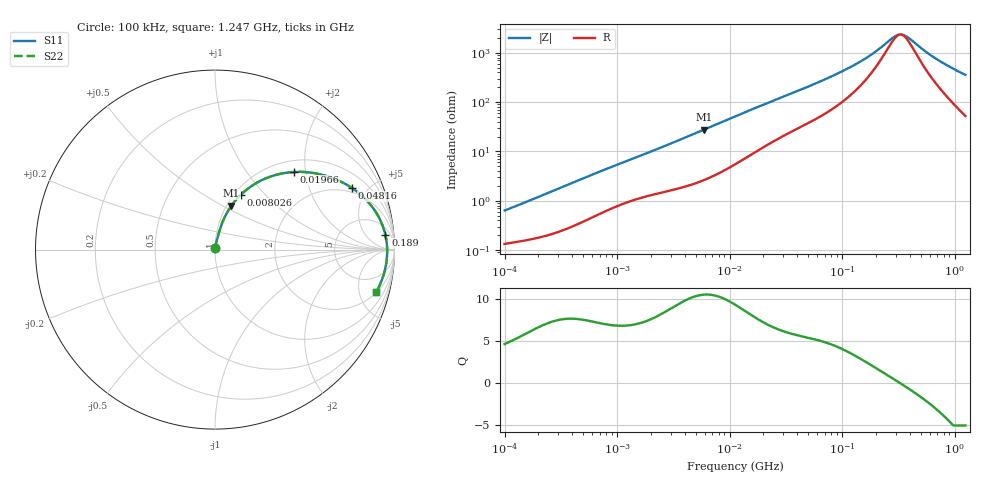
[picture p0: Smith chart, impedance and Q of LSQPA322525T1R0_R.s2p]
! LSQPA322525T1R0_R  S-PARAMETER MODEL  ( General Type )
! Model Generated by TAIYO YUDEN Corporation (http://www.ty-top.com)
! Version 2.0
! TAIYO YUDEN Control No. 100810NF25SB-FKC
! Copyright(c) 2007 TAIYO YUDEN CO.,LTD. All Rights Reserved.
! Product Description (link to TY-COMPAS)
! https://ds.yuden.co.jp/TYCOMPAS/or/detail?pn=LSQPA322525T1R0MR&u=M
! Products Name : Inductors
! Characteristics :
!  Inductance : 1.0 uH , SRF(min) : 250 MHz , DC Resistance(max) : 0.0715 Ohm
!  Rated Current : Saturation :2000 mA , Temp Rise : 1440 mA (40 degC)
!  Case Size : 3.2 x 2.5 / 0.126 x 0.098 [mm/inch] , Thickness : 2.5 / 0.098 [mm/inch]
!  (Conditions: Temperature = 25 degC , DC Bias Current/Voltage = 0A / 0V)
! External Node Assignments :
!  1  o---GGG---o  2
! GND o---------o GND
! Frequency Range : 0.1MHz  -  1246.521536MHz  [ 402 STEP ]
# MHz S RI R 50
! Freq[MHz].  S11 Real  S11 Imag  S21 Real  S21 Imag  S12 Real  S12 Imag  S22 Real  S22 Imag
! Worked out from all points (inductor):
!   401 points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, 100 kHz to 1.247 GHz, reference 50 ohm
!   read as one part in series: L = 967 nH near 104.8 kHz
!   highest Q = 10.5 at 5.907 MHz (marker M1), where L = 743 nH
!   self-resonance near 329.6 MHz
!   S11 on the Smith chart (normalised r, x): 100 kHz: 1.00, +0.01; 8.026 MHz: 1.07, +0.74; 19.66 MHz: 1.24, +1.73; 48.16 MHz: 1.72, +3.93; 189 MHz: 10, +18; 1.247 GHz: 2.05, -7.07
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0.1  0.00137 0.00618  0.9986 -0.00618  0.9986 -0.00618  0.00137 0.00618
0.485322  0.00439 0.0274  0.9956 -0.0274  0.9956 -0.0274  0.00439 0.0274
1.188834  0.0127 0.0607  0.9873 -0.0607  0.9873 -0.0607  0.0127 0.0607
2.355372  0.0265 0.1101  0.9735 -0.1101  0.9735 -0.1101  0.0265 0.1101
5.907315  0.0913 0.2443  0.9087 -0.2443  0.9087 -0.2443  0.0913 0.2443
8.026023  0.1448 0.3066  0.8552 -0.3066  0.8552 -0.3066  0.1448 0.3066
11.16477  0.2317 0.3717  0.7683 -0.3717  0.7683 -0.3717  0.2317 0.3717
19.66038  0.4417 0.4326  0.5583 -0.4326  0.5583 -0.4326  0.4417 0.4326
29.35345  0.5998 0.4161  0.4002 -0.4161  0.4002 -0.4161  0.5998 0.4161
48.15965  0.7619 0.344  0.2381 -0.344  0.2381 -0.344  0.7619 0.344
54.18507  0.7928 0.3216  0.2072 -0.3216  0.2072 -0.3216  0.7928 0.3216
77.17353  0.8666 0.2498  0.1334 -0.2498  0.1334 -0.2498  0.8666 0.2498
109.915  0.9137 0.1785  0.0863 -0.1785  0.0863 -0.1785  0.9137 0.1785
145.8573  0.9365 0.1263  0.0635 -0.1263  0.0635 -0.1263  0.9365 0.1263
189.0427  0.9491 0.083  0.0509 -0.083  0.0509 -0.083  0.9491 0.083
262.9719  0.9573 0.0328  0.0427 -0.0328  0.0427 -0.0328  0.9573 0.0328
310.1588  0.959 0.00878  0.041 -0.00878  0.041 -0.00878  0.959 0.00878
332.8908  0.9593 -0.00144  0.0407 0.00144  0.0407 0.00144  0.9593 -0.00144
357.2889  0.9594 -0.0117  0.0406 0.0117  0.0406 0.0117  0.9594 -0.0117
675.2729  0.9473 -0.1117  0.0527 0.1117  0.0527 0.1117  0.9473 -0.1117
939.3529  0.9275 -0.1752  0.0725 0.1752  0.0725 0.1752  0.9275 -0.1752
1246.522  0.8972 -0.2385  0.1028 0.2385  0.1028 0.2385  0.8972 -0.2385
